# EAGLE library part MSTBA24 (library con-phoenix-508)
PHOENIX
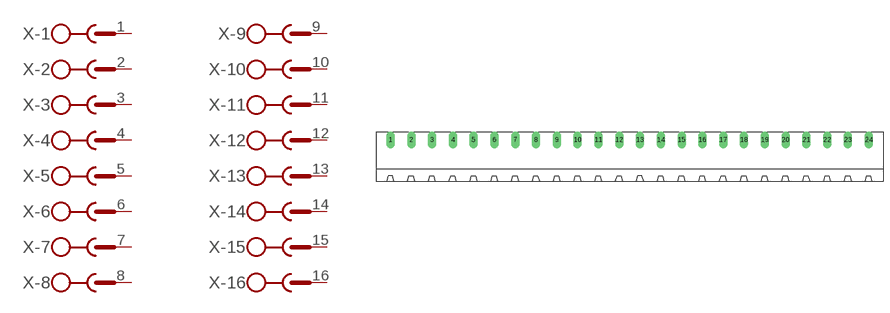
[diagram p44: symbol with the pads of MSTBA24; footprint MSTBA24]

Designator prefix X; gates -1=SK -2=SK -3=SK -4=SK -5=SK -6=SK -7=SK -8=SK -9=SK -10=SK -11=SK -12=SK -13=SK -14=SK -15=SK -16=SK -17=SK -18=SK -19=SK -20=SK -21=SK -22=SK -23=SK -24=SKV

## MSTBA24 (OC_FARNELL: unknown; OC_NEWARK: unknown)  [MSTBA24]
1  -1:1  pas
2  -2:1  pas
3  -3:1  pas
4  -4:1  pas
5  -5:1  pas
6  -6:1  pas
7  -7:1  pas
8  -8:1  pas
9  -9:1  pas
10  -10:1  pas
11  -11:1  pas
12  -12:1  pas
13  -13:1  pas
14  -14:1  pas
15  -15:1  pas
16  -16:1  pas
17  -17:1  pas
18  -18:1  pas
19  -19:1  pas
20  -20:1  pas
21  -21:1  pas
22  -22:1  pas
23  -23:1  pas
24  -24:1  pas

## Footprint MSTBA24 (pad centres in mm)
PHOENIX
drill 1.397 long: 1 -58.42,5.08; 2 -53.34,5.08; 3 -48.26,5.08; 4 -43.18,5.08; 5 -38.1,5.08; 6 -33.02,5.08; 7 -27.94,5.08; 8 -22.86,5.08; 9 -17.78,5.08; 10 -12.7,5.08; 11 -7.62,5.08; 12 -2.54,5.08; 13 2.54,5.08; 14 7.62,5.08; 15 12.7,5.08; 16 17.78,5.08; 17 22.86,5.08; 18 27.94,5.08; 19 33.02,5.08; 20 38.1,5.08; 21 43.18,5.08; 22 48.26,5.08; 23 53.34,5.08; 24 58.42,5.08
